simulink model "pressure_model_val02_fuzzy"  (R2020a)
settings: Solver=VariableStepAuto  StartTime=0.0  StopTime=tfin  RelTol=1e-3
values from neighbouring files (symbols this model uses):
  Ts = 5    [sisopres.m]
undefined symbols (not defined in the file or in its folder): magnitude
libraries: fuzblock x1

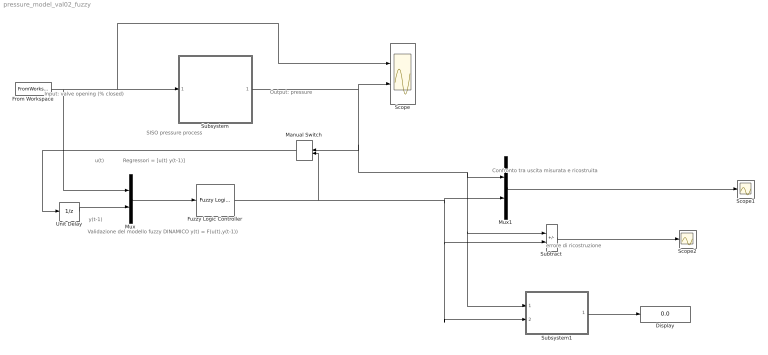
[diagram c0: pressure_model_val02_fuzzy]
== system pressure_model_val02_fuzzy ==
  note: Confronto tra uscita misurata e ricostruita
  note: Regressori = [u(t) y(t-1)]
  note: y(t-1)
  note: u(t)
  note: Validazione del modello fuzzy DINAMICO y(t) = F(u(t),y(t-1))
  note: Output: pressure
  note: Input: valve opening (% closed)
  note: SISO pressure process
  note: errore di ricostruzione
  Display : Display
  From Workspace : FromWorkspace  VariableName=[tsim U]  SampleTime=Ts
  Fuzzy Logic Controller : fuzblock/Fuzzy Logic  Controller  FIS=FIS02  OutputSampleNumber=101  DataType=double  FuzzifiedInputs=off  RuleFiringStrengths=off  RuleOutputs=off  AggregatedOutputs=off  SimulateUsing=Interpreted execution  OutOfRangeInputValueMessage=warning  NoRuleFiredMessage=warning  EmptyOutputFuzzySetMessage=warning
  Manual Switch : ManualSwitch
  Mux : Mux  Inputs=2
  Mux1 : Mux  Inputs=2
  Scope : Scope  NumInputPorts=2
  Scope1 : Scope
  Scope2 : Scope
  Subsystem : Subsystem
  Subsystem1 : Subsystem
  Subtract : Sum  Inputs=+-
  Unit Delay : UnitDelay  SampleTime=Ts  HasFrameUpgradeWarning=on
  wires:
  From Workspace/1 -> Mux/1, Scope/1, Subsystem/1(u)
  Mux/1 -> Fuzzy Logic Controller/1
  Subsystem1/1(VAF%) -> Display/1
  Subtract/1 -> Scope2/1
  Subsystem/1(y) -> Manual Switch/1, Subsystem1/1(y_mis), Subtract/1, Mux1/1, Scope/2
  Fuzzy Logic Controller/1 -> Manual Switch/2, Subsystem1/2(y_prev), Subtract/2, Mux1/2
  Mux1/1 -> Scope1/1
  Manual Switch/1 -> Unit Delay/1
  Unit Delay/1 -> Mux/2

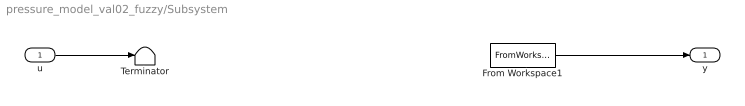
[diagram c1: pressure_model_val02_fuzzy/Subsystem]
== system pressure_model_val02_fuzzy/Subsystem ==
  u : Inport
  From Workspace1 : FromWorkspace  VariableName=[tsim Y]  SampleTime=Ts
  Terminator : Terminator
  y : Outport
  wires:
  From Workspace1/1 -> y/1
  u/1 -> Terminator/1

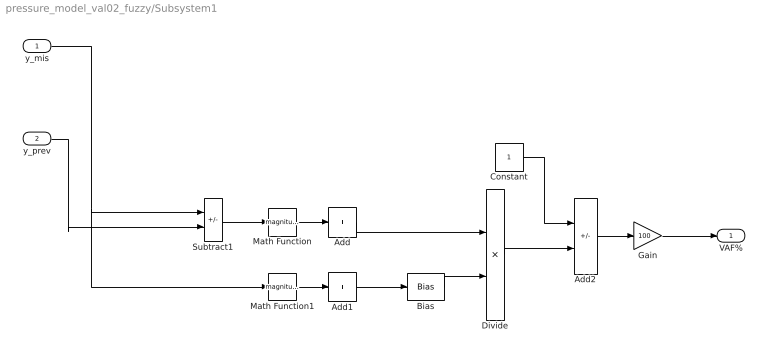
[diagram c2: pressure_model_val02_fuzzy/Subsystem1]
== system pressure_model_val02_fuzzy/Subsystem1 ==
  y_mis : Inport
  y_prev : Inport  Port=2
  Add : Sum  Inputs=+
  Add1 : Sum  Inputs=+
  Add2 : Sum  Inputs=+-
  Bias : Bias  Bias=1e-7
  Constant : Constant
  Divide : Product  Inputs=*/
  Gain : Gain  Gain=100
  Math Function : Math  Operator=magnitude^2
  Math Function1 : Math  Operator=magnitude^2
  Subtract1 : Sum  Inputs=+-
  VAF% : Outport
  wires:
  Add2/1 -> Gain/1
  Math Function/1 -> Add/1
  Bias/1 -> Divide/2
  y_mis/1 -> Math Function1/1, Subtract1/1
  Add1/1 -> Bias/1
  Math Function1/1 -> Add1/1
  Subtract1/1 -> Math Function/1
  Constant/1 -> Add2/1
  Divide/1 -> Add2/2
  Add/1 -> Divide/1
  y_prev/1 -> Subtract1/2
  Gain/1 -> VAF%/1
